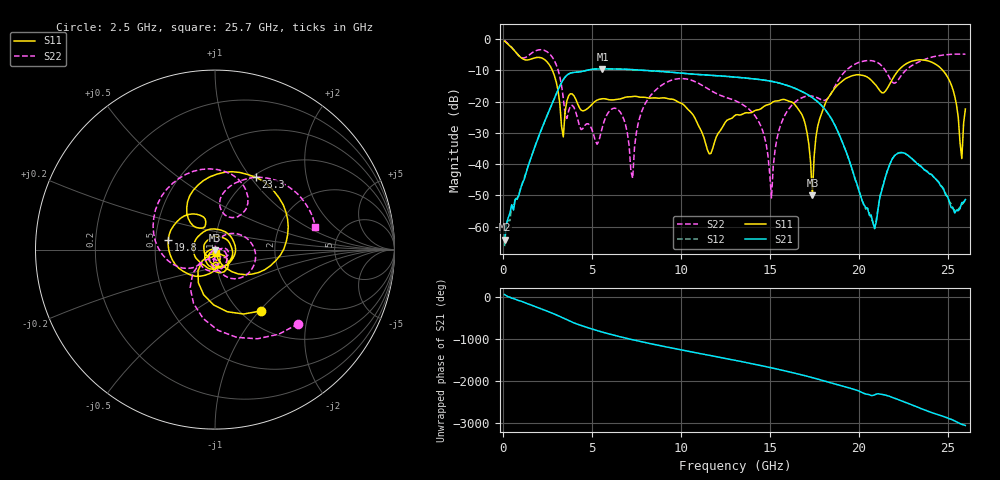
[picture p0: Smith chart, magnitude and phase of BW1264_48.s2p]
!Keysight Technologies,N5245B,MY57181159,A.13.60.06
!Date: Friday, December 18, 2020 23:54:35
!Correction: S11(Full 2 Port(1,2))
!S21(Full 2 Port(1,2))
!S12(Full 2 Port(1,2))
!S22(Full 2 Port(1,2))
!S2P File: Measurements: S11, S21, S12, S22:
# Hz S  dB  R 50
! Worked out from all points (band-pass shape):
!   260 points, 100 MHz to 26 GHz, reference 50 ohm
!   highest |S21| = -9.54 dB at 5.6 GHz (marker M1); lowest = -64.2 dB at 100 MHz (marker M2)
!   |S21| within 3 dB of the highest: 3.453 GHz to 13.78 GHz (10.33 GHz wide, 120 % of centre)
!   lowest |S11| = -50.0 dB at 17.4 GHz (marker M3), VSWR 1.01, Z = 49.9 - j0.3 ohm
!   |S11| at or under -10 dB: 2.781 GHz to 22.24 GHz (19.46 GHz wide, 156 % of centre); 24.73 GHz to end of sweep
!   |S22| runs from -50.8 to -0.5 dB; largest |S21 - S12| = 0.00076
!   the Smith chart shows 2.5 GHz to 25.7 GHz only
!   S11 on the Smith chart (normalised r, x): 2.5 GHz: 1.22, -1.02; 19.8 GHz: 0.58, +0.07; 23.3 GHz: 1.03, +1.06; 25.7 GHz: 1.01, -0.04
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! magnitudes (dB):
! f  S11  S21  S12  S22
! 100 MHz  -0.7  -64.2  -66.2  -0.5
! 2.5 GHz  -7.4  -24.3  -24.3  -4.1
! 3.4 GHz  -31.3  -13.0  -13.0  -18.9
! 4.5 GHz  -23.0  -10.3  -10.3  -28.6
! 5.6 GHz  -19.1  -9.5  -9.5  -28.1
! 6.6 GHz  -19.1  -9.6  -9.6  -23.4
! 7.3 GHz  -18.4  -9.8  -9.8  -44.5
! 8.8 GHz  -18.9  -10.3  -10.3  -15.3
! 11.6 GHz  -36.7  -11.6  -11.6  -16.1
! 13.1 GHz  -24.2  -12.2  -12.2  -19.8
! 14.6 GHz  -21.9  -13.1  -13.1  -29.2
! 15.1 GHz  -20.5  -13.5  -13.5  -50.8
! 15.6 GHz  -19.6  -14.2  -14.2  -27.7
! 16.8 GHz  -24.0  -16.7  -16.7  -18.8
! 17.4 GHz  -50.0  -18.7  -18.7  -18.3
! 18 GHz  -22.5  -21.8  -21.8  -19.6
! 19.8 GHz  -11.5  -45.0  -44.6  -8.0
! 20.9 GHz  -14.3  -60.5  -60.6  -7.2
! 21.7 GHz  -14.9  -40.9  -40.7  -12.0
! 23.3 GHz  -6.7  -39.9  -39.7  -7.5
! 25.7 GHz  -33.2  -54.2  -53.7  -4.8
! 26 GHz  -22.4  -51.3  -51.3  -4.8
